FUNCTION_BLOCK Immediate_Stop_DUT

VAR_IN_OUT
    SD_SMD_IO: DUT_AMCI_Stepper;
END_VAR	

VAR_INPUT
			
END_VAR

VAR_OUTPUT
	Enable: BOOL;
	Error: BOOl;
END_VAR

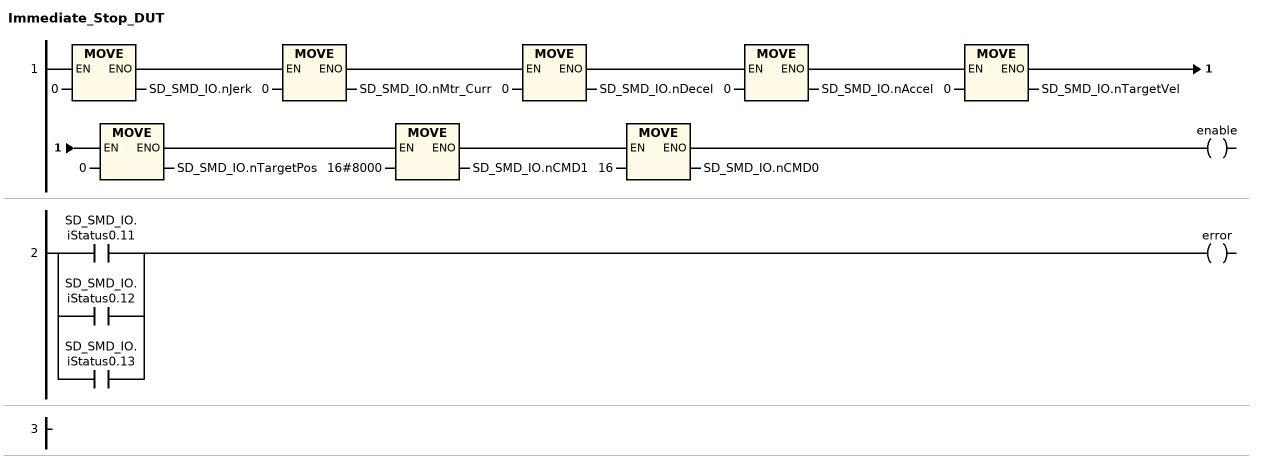
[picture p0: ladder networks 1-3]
// NETWORK 1
SD_SMD_IO.nJerk := 0;
SD_SMD_IO.nMtr_Curr := 0;
SD_SMD_IO.nDecel := 0;
SD_SMD_IO.nAccel := 0;
SD_SMD_IO.nTargetVel := 0;
SD_SMD_IO.nTargetPos := 0;
SD_SMD_IO.nCMD1 := 16#8000;
SD_SMD_IO.nCMD0 := 16;
enable := TRUE;

// NETWORK 2
error := SD_SMD_IO.iStatus0.11 OR SD_SMD_IO.iStatus0.12 OR SD_SMD_IO.iStatus0.13;

// NETWORK 3

END_FUNCTION_BLOCK
